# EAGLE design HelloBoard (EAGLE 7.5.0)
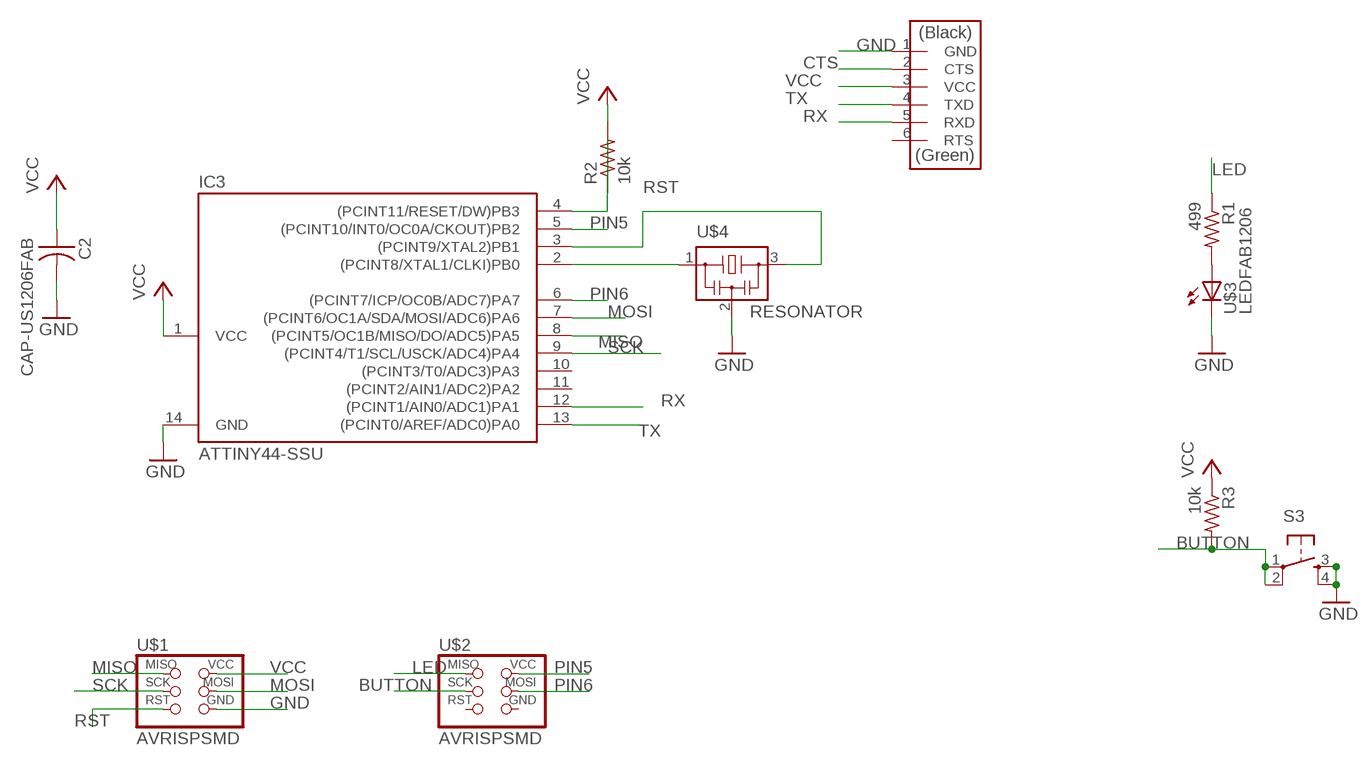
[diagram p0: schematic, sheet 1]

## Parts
C2  CAP-US1206FAB  [C1206FAB]
IC3  ATTINY44-SSU  [SOIC14]
R1  499  RES-US1206FAB  [R1206FAB]
R2  10k  RES-US1206FAB  [R1206FAB]
R3  10k  RES-US1206  [R1206]
S3  6MM_SWITCH6MM_SWITCH  [6MM_SWITCH]
U$1  AVRISPSMD  [2X03SMD]
U$2  AVRISPSMD  [2X03SMD]
U$3  LEDFAB1206  [LED1206FAB]
U$4  RESONATOR  [EFOBM]
U$5  FTDI-SMD-HEADER  [1X06SMD]

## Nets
BUTTON: R3.2 S3.1(P) S3.2(P1) U$2.3(SCK)
CTS: U$5.2(CTS)
GND: C2.2 IC3.14(GND) S3.3(S) S3.4(S1) U$1.6(GND) U$3.2(C) U$4.2 U$5.1(GND)
LED: R1.1 U$2.1(MISO)
MISO: IC3.8((PCINT5/OC1B/MISO/DO/ADC5)PA5) U$1.1(MISO)
MOSI: IC3.7((PCINT6/OC1A/SDA/MOSI/ADC6)PA6) U$1.4(MOSI)
N$1: R1.2 U$3.1(A)
N$2: IC3.3((PCINT9/XTAL2)PB1) U$4.3
N$3: IC3.2((PCINT8/XTAL1/CLKI)PB0) U$4.1
PIN5: IC3.5((PCINT10/INT0/OC0A/CKOUT)PB2) U$2.2(VCC)
PIN6: IC3.6((PCINT7/ICP/OC0B/ADC7)PA7) U$2.4(MOSI)
RST: IC3.4((PCINT11/RESET/DW)PB3) R2.1 U$1.5(RST)
RX: IC3.12((PCINT1/AIN0/ADC1)PA1) U$5.5(RXD)
SCK: IC3.9((PCINT4/T1/SCL/USCK/ADC4)PA4) U$1.3(SCK)
TX: IC3.13((PCINT0/AREF/ADC0)PA0) U$5.4(TXD)
VCC: C2.1 IC3.1(VCC) R2.2 R3.1 U$1.2(VCC) U$5.3(VCC)
Unconnected: IC3.10((PCINT3/T0/ADC3)PA3) IC3.11((PCINT2/AIN1/ADC2)PA2) U$2.5(RST) U$2.6(GND) U$5.6(RTS)

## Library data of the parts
C2 = fab:CAP-US
IC3 = fab:ATTINY44
R1-R3 = fab:RES-US: Resistor (US Symbol)
S3 = fab:6MM_SWITCH: OMRON SWITCH
U$1 U$2 = fab:AVRISP
U$3 = fab:LED: LED
U$4 = fab:RESONATOR
U$5 = fab:FTDI-SMD-HEADER

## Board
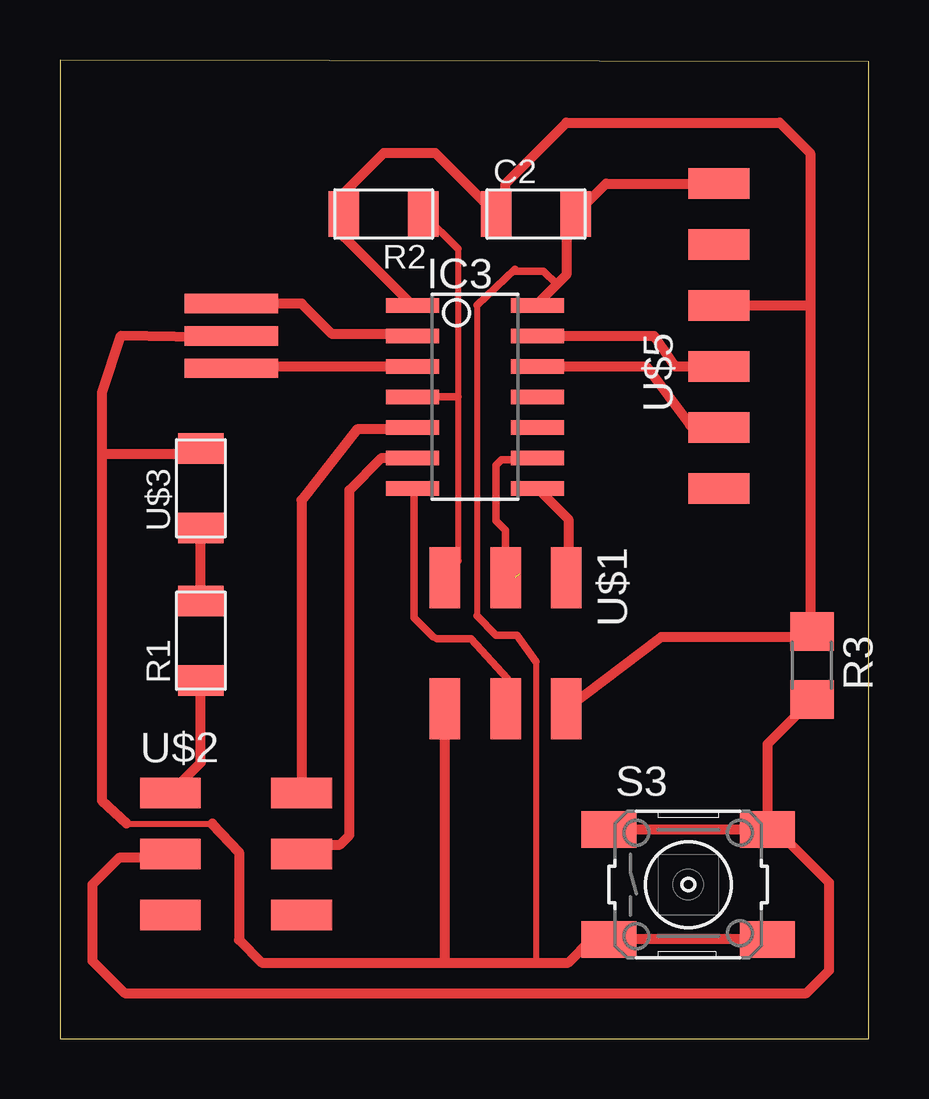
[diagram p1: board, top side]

Size 33.71 x 40.79 mm. Coordinates in mm from the lower left corner, seen from the top.
Outline: 0,0 33.71,0 33.71,40.71 0,40.79 0,0
Copper layers (1*16): Top 0.035mm / dielectric 1.5mm / Bottom 0.035mm
Design rules "default": minimum track width 10mil, minimum drill 24mil, track to track 8mil, track to pad 8mil, pad to pad 8mil, via to via 8mil, smd to smd 8mil, copper to edge 40mil, drill to drill 8mil, minimum pad ring 10mil, minimum via ring 8mil, stop-mask expansion 4mil, vias tented up to drill 0mil, thermal gap 10mil

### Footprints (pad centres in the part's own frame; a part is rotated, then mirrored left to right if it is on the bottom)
C1206FAB = smd 1.27 x 1.905: 1 -1.651,0; 2 1.651,0
SOIC14 = smd 0.61 x 2.21: 1 -3.81,-2.603; 2 -2.54,-2.603; 3 -1.27,-2.603; 4 0,-2.603; 5 1.27,-2.603; 6 2.54,-2.603; 7 3.81,-2.603; 8 3.81,2.603; 9 2.54,2.603; 10 1.27,2.603; 11 0,2.603; 12 -1.27,2.603; 13 -2.54,2.603; 14 -3.81,2.603
R1206FAB = smd 1.27 x 1.905: 1 -1.651,0; 2 1.651,0
R1206 = smd 1.6 x 1.803: 1 -1.422,0; 2 1.422,0
6MM_SWITCH = smd 2.286 x 1.524: 1 -3.302,2.286; 2 3.302,2.286; 3 -3.302,-2.286; 4 3.302,-2.286
2X03SMD = smd 2.54 x 1.27: 1 -2.54,2.54; 2 2.92,2.54; 3 -2.54,0; 4 2.92,0; 5 -2.54,-2.54; 6 2.92,-2.54
LED1206FAB = smd 1.27 x 1.905: 1 -1.651,0; 2 1.651,0
EFOBM = smd 0.8 x 3.9: 1 -1.35,0; 2 0,0; 3 1.35,0
1X06SMD = smd 2.54 x 1.27: 1 0,6.35; 2 0,3.81; 3 0,1.27; 4 0,-1.27; 5 0,-3.81; 6 0,-6.35

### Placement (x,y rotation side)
C2  19.84,34.37 0 top
IC3  17.3,26.75 270 top
R1  5.87,16.59 90 top
R2  13.49,34.37 180 top
R3  31.35,15.56 270 top
S3  26.19,6.43 0 top
U$1  18.57,16.67 270 top
U$2  7.14,7.7 0 top
U$3  5.87,22.94 90 top
U$4  7.14,29.29 270 top
U$5  27.46,29.29 0 top

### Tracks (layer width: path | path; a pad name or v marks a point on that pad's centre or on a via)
BUTTON
  Top 0.406: S3.2 S3.1 | R3.2 29.5,12.28 S3.2 | U$2.3 4.45,7.54 2.46,7.54 1.35,6.43 1.35,3.25 2.7,1.91 31.11,1.91 32.07,2.86 32.07,6.51 29.86,8.71 S3.2
GND
  Top 0.254: 2.78,8.97 6.35,8.97 | 19.84,15.72 19.84,3.17 | 17.38,30.56 17.38,17.62
  Top 0.305: 20.72,31.43 20.16,31.99 18.97,31.99 18.97,32.07 17.38,30.56 | 17.38,17.62 18.18,16.83 19.05,16.83 19.84,15.72
  Top 0.406: U$5.1 22.77,35.64 C2.2 21.11,33.99 21.11,31.83 20.72,31.43 19.91,30.62 IC3.14 | S3.4 S3.3 22.16,4.14 21.19,3.17 19.84,3.17 16.03,3.17 | U$4.2 7.06,29.21 2.54,29.29 1.75,26.91 1.75,24.37 | 1.75,24.37 1.75,9.92 2.78,8.97 | 6.35,8.97 7.46,7.78 7.46,4.13 8.41,3.17 16.03,3.17 | U$3.2 5.65,24.37 1.75,24.37 | U$1.6 16.03,3.17
LED
  Top 0.406: U$2.1 5.87,11.51 R1.1
MISO
  Top 0.406: IC3.8 21.19,21.65 21.19,20.4 21.11,20.32 U$1.1
MOSI
  Top 0.305: IC3.7 14.76,22.88 14.76,17.54 15.56,16.75 15.72,16.67 17.14,16.67 18.65,15 18.65,14.29 18.57,14.21 U$1.4
N$1
  Top 0.406: R1.2 U$3.1
N$2
  Top 0.406: U$4.3 7.22,28.02 IC3.3
N$3
  Top 0.406: IC3.2 14.62,29.37 11.35,29.37 10.08,30.64 U$4.1
PIN5
  Top 0.406: IC3.5 14.62,25.4 12.38,25.4 10.06,22.45 U$2.2
PIN6
  Top 0.406: U$2.4 10.46,8.1 11.67,8.1 12.06,8.49 12.06,22.86 13.41,24.21 IC3.6
RST
  Top 0.254: 16.59,32.92 16.59,26.75 16.59,19.92
  Top 0.305: R2.1 16.59,32.92 | 16.59,19.92 16.03,19.37 U$1.5 | 16.59,26.75 IC3.4
RX
  Top 0.406: IC3.12 24.45,28.02 26.27,25.56 26.99,25.56 27.07,25.48 U$5.5
SCK  (1 unrouted)
  Top 0.305: 19.83,24.13 19.75,24.05 19.67,24.13 18.41,24.13 18.18,23.89 18.18,21.59 18.57,21.19 U$1.3 18.97,19.21
  Top 0.406: IC3.9 19.83,24.13
TX
  Top 0.406: IC3.13 24.77,29.29 25.64,28.02 U$5.4
VCC
  Top 0.406: IC3.1 11.84,33.42 R2.2 11.84,35.26 13.49,36.91 15.65,36.91 C2.1 18.57,34.75 18.57,35.64 21.11,38.18 30,38.18 31.27,36.91 31.27,30.56 | 31.27,30.56 31.27,17.06 | U$5.3 31.27,30.56 | R3.1 31.27,17.06 | 31.27,17.06 30.96,16.74 25.06,16.74 U$1.2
